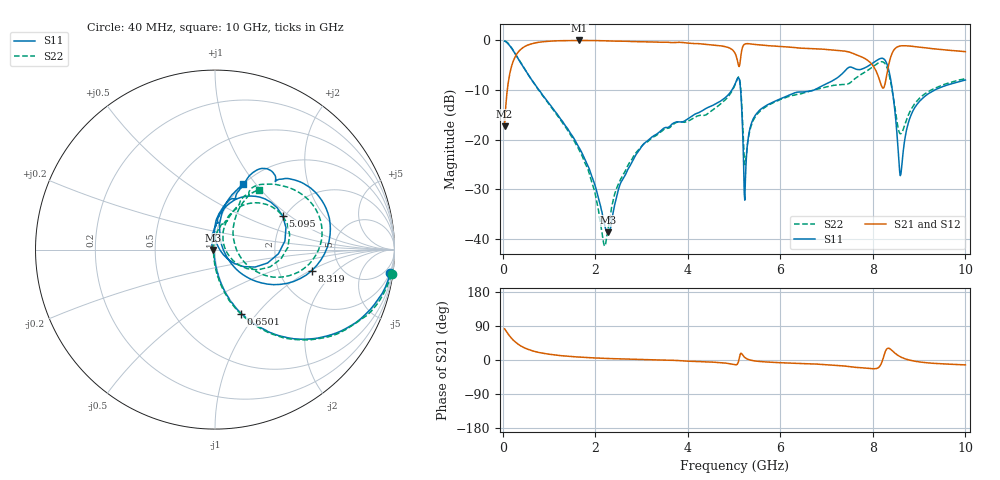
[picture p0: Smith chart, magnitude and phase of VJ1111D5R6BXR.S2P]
! VJ1111D5R6BXR
! DATE 03/04/2022  14:19
! CAPACITORS MOUNTED IN SERIES ON 25 MIL THICK MICROSTRIP SUBSTRATE
# GHz  S  MA  R  50.00
!  FREQ  S11M  S11A  S21M  S21A  S12M  S12A  S22M  S22A
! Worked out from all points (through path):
!   801 points, 40 MHz to 10 GHz, reference 50 ohm
!   highest |S21| = 0.00 dB at 1.659 GHz (marker M1); lowest = -17.4 dB at 40 MHz (marker M2)
!   group delay of S21, straight-line fit = 9.78 ps
!   lowest |S11| = -38.8 dB at 2.281 GHz (marker M3), VSWR 1.02, Z = 48.9 - j0.206 ohm
!   |S11| at or under -10 dB: 780.3 MHz to 4.954 GHz (4.174 GHz wide, 146 % of centre); 5.141 GHz to 6.73 GHz (1.589 GHz wide, 26.8 % of centre); 8.421 GHz to 9.339 GHz (918 MHz wide, 10.3 % of centre)
!   |S22| runs from -41.5 to -0.1 dB; largest |S21 - S12| = 0.009
!   S11 on the Smith chart (normalised r, x): 40 MHz: 2, -15; 650 MHz: 0.99, -0.83; 5.095 GHz: 1.95, +0.88; 8.319 GHz: 3.07, -1.04; 10 GHz: 0.99, +0.86
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0.04  0.9837 -7.7  0.1355 82.1  0.1359 81.7  0.9941 -8.0
0.2392  0.7717 -39.1  0.639 51.0  0.6392 51.4  0.7761 -39.4
0.65005  0.385 -67.8  0.9322 23.9  0.9358 23.6  0.3836 -68.2
1.6585  0.08187 -88.3  0.9996 7.7  1.003 7.6  0.07717 -91.6
1.7083  0.07359 -89.3  0.9987 7.3  1.004 7.2  0.06915 -92.4
2.1814  0.01514 -122.5  0.9923 4.4  0.9964 4.2  0.0089 -156.8
2.281  0.01152 -169.4  0.9888 3.9  0.9934 3.7  0.01273 128.7
2.7043  0.04988 109.2  0.979 2.2  0.9832 2.1  0.05456 92.0
3.36415  0.1169 91.9  0.9604 0.0  0.9649 -0.1  0.1141 80.8
5.02  0.3616 55.6  0.7439 -12.4  0.7468 -12.5  0.3568 46.8
5.0947  0.421 26.3  0.5624 -4.6  0.5646 -4.7  0.4276 19.7
5.2441  0.03832 77.4  0.9239 5.5  0.9276 5.4  0.05638 29.1
5.35615  0.1361 89.6  0.9227 -0.4  0.9257 -0.5  0.1312 67.4
5.518  0.1899 84.7  0.9041 -3.5  0.9079 -3.6  0.1845 67.1
6.6883  0.3112 68.5  0.8251 -10.3  0.8283 -10.4  0.3122 62.3
7.99555  0.5892 41.2  0.561 -23.2  0.5631 -23.3  0.5402 39.5
8.2072  0.6606 15.4  0.3334 -1.5  0.335 -1.7  0.6088 12.9
8.31925  0.5516 -12.3  0.5014 30.8  0.5032 30.6  0.5098 -11.6
8.34415  0.501 -18.8  0.5723 30.9  0.5758 30.8  0.4639 -16.9
8.6056  0.04482 33.4  0.8811 7.7  0.8843 7.6  0.1147 18.7
8.96665  0.23 78.2  0.8604 -4.4  0.864 -4.5  0.2493 59.3
10  0.3983 67.3  0.7701 -12.9  0.7733 -13.1  0.4115 53.9
